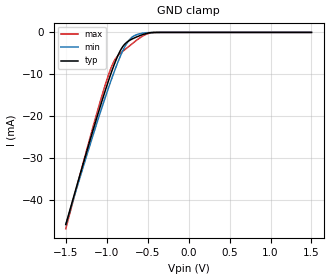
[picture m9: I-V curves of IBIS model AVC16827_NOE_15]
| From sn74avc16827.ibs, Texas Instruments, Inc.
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[Model]   AVC16827_NOE_15
Model_type  Input
Vinl=0.8
Vinh=1.0
| variable   typ   min   max
C_comp   2.32pF   1.53pF   2.68pF
[Temperature Range]   40   100   -40
| Ambient temperature   25   85   -40
[Voltage range]   1.5   1.4   1.6
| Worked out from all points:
|   GND clamp passes 1 mA (typ) near -0.62 V on its own axis
[GND Clamp]
| AVC16827_NOE_15
|   Voltage   I(typ)   I(min)   I(max)
-1.5V     -45.76mA   -45.79mA   -46.75mA
-1.16V    -22.81mA   -24.04mA   -21.97mA
-1.05V    -15.81mA   -17.35mA   -14.51mA
-970mV    -11.02mA   -12.71mA   -9.647mA
-900mV    -7.224mA   -8.898mA   -6.51mA
-825mV    -4.016mA   -5.248mA   -4.839mA
-755mV    -2.351mA   -2.59mA    -3.725mA
-690mV    -1.576mA   -1.13mA    -2.715mA
-630mV    -1.046mA   -515.2uA   -1.785mA
-545mV    -431.5uA   -137.4uA   -708.8uA
-430mV    -25.26uA   -18.03uA   -33.69uA
1.5V      251.2pA    918pA      12.88pA
